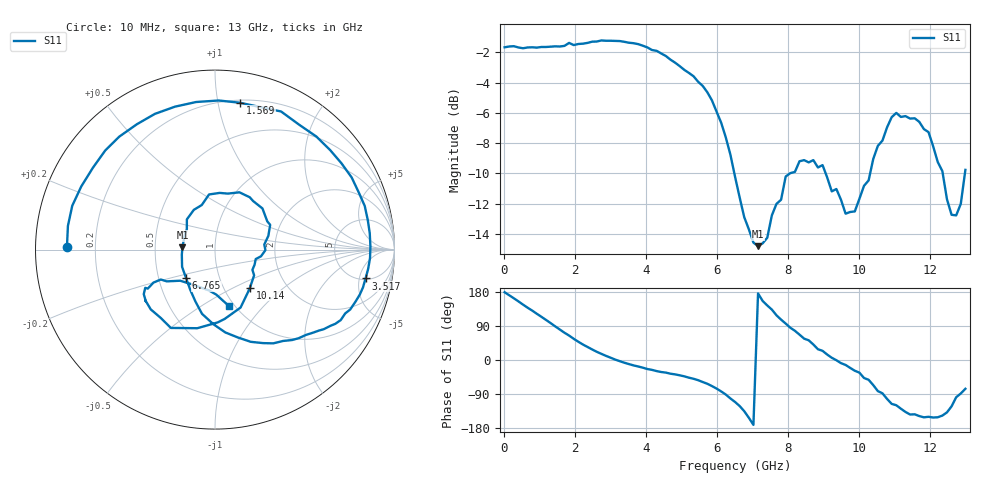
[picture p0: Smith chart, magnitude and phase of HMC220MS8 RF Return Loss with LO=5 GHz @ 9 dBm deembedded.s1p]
!Hittite Microwave Corporation
!12 Elizabeth Drive
!Chelmsford, MA 01824
!Tel: 978-250-3343
!Fax: 978-250-3373
!Device: HMC220MS8, 5-12 GHz, GaAS MMIC SMT Double-Balanced Mixer in 8-lead MSOP package
!Misc: RF Return Loss, LO = 5 GHz @ 9dBm, Room
# MHZ S MA R 50
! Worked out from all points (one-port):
!   101 points, 10 MHz to 13 GHz, reference 50 ohm
!   lowest |S11| = -14.8 dB at 7.154 GHz (marker M1), VSWR 1.44, Z = 34.6 + j0.969 ohm
!   |S11| at or under -10 dB: 6.487 GHz to 8.051 GHz (1.564 GHz wide, 21.5 % of centre); 9.062 GHz to 10.31 GHz (1.252 GHz wide, 12.9 % of centre); 12.36 GHz to 12.99 GHz (624.8 MHz wide, 4.93 % of centre)
!   S11 on the Smith chart (normalised r, x): 10 MHz: 0.10, +0.01; 1.569 GHz: 0.22, +1.16; 3.517 GHz: 5.22, -6.20; 6.765 GHz: 0.69, -0.23; 10.14 GHz: 1.32, -0.61; 13 GHz: 0.94, -0.67
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10  0.825 178.9
399.7  0.824 154.7
919.3  0.823 121.9
1568.8  0.83 80.3
1698.7  0.834 71.9
2088.4  0.846 48.1
2478.1  0.861 27.8
3257.5  0.865 -3.1
3517.3  0.854 -10.8
4296.7  0.803 -29.3
4946.2  0.715 -40.4
5855.5  0.551 -68.8
6505  0.309 -110.7
6764.8  0.227 -135.0
7154.5  0.182 175.7
7544.2  0.23 133.0
8193.7  0.32 77.1
8973.1  0.337 24.2
9752.5  0.236 -20.9
10142.2  0.288 -47.5
10402  0.353 -66.2
10791.7  0.449 -102.7
11051.5  0.501 -119.4
11441.2  0.48 -143.9
11960.8  0.433 -149.9
12610.3  0.231 -122.3
12870.1  0.251 -88.3
13000  0.325 -76.0
